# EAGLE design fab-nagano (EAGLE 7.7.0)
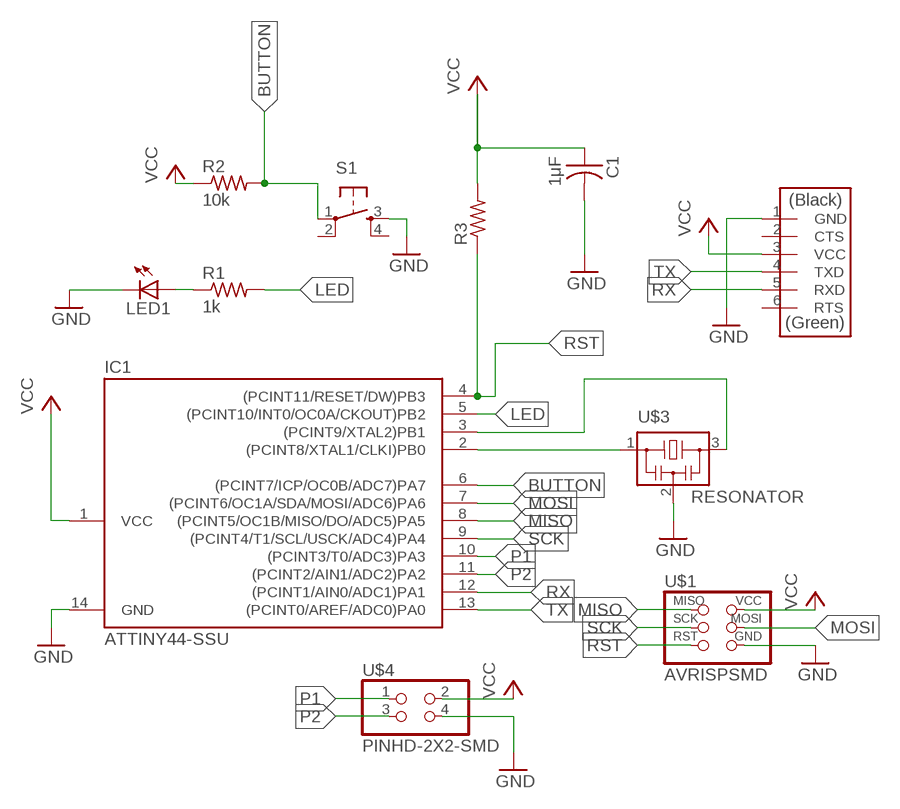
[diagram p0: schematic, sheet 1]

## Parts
C1  1μF  CAP-US1206FAB  [C1206FAB]
IC1  ATTINY44-SSU  [SOIC14]
LED1  LEDCHIP-LED0805  [CHIP-LED0805]
R1  1k  RES-US1206FAB  [R1206FAB]
R2  10k  RES-US1206FAB  [R1206FAB]
R3  RES-US1206FAB  [R1206FAB]
S1  6MM_SWITCH6MM_SWITCH  [6MM_SWITCH]
U$1  AVRISPSMD  [2X03SMD]
U$2  FTDI-SMD-HEADER  [1X06SMD]
U$3  RESONATOR  [EFOBM]
U$4  PINHD-2X2-SMD  [2X02SMD]

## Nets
BUTTON: IC1.6((PCINT7/ICP/OC0B/ADC7)PA7) R2.2 S1.1(P)
GND: C1.2 IC1.14(GND) LED1.C S1.3(S) U$1.6(GND) U$2.1(GND) U$3.2 U$4.4
LED: IC1.5((PCINT10/INT0/OC0A/CKOUT)PB2) R1.2
MISO: IC1.8((PCINT5/OC1B/MISO/DO/ADC5)PA5) U$1.1(MISO)
MOSI: IC1.7((PCINT6/OC1A/SDA/MOSI/ADC6)PA6) U$1.4(MOSI)
N$1: LED1.A R1.1
N$2: IC1.2((PCINT8/XTAL1/CLKI)PB0) U$3.1
N$3: IC1.3((PCINT9/XTAL2)PB1) U$3.3
P1: IC1.10((PCINT3/T0/ADC3)PA3) U$4.1
P2: IC1.11((PCINT2/AIN1/ADC2)PA2) U$4.3
RST: IC1.4((PCINT11/RESET/DW)PB3) R3.1 U$1.5(RST)
RX: IC1.12((PCINT1/AIN0/ADC1)PA1) U$2.5(RXD)
SCK: IC1.9((PCINT4/T1/SCL/USCK/ADC4)PA4) U$1.3(SCK)
TX: IC1.13((PCINT0/AREF/ADC0)PA0) U$2.4(TXD)
VCC: C1.1 IC1.1(VCC) R2.1 R3.2 U$1.2(VCC) U$2.3(VCC) U$4.2
Unconnected: S1.2(P1) S1.4(S1) U$2.2(CTS) U$2.6(RTS)

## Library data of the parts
C1 = fab:CAP-US
IC1 = fab:ATTINY44
LED1 = led:LED: LED
R1-R3 = fab:RES-US: Resistor (US Symbol)
S1 = fab:6MM_SWITCH: OMRON SWITCH
U$1 = fab:AVRISP
U$2 = fab:FTDI-SMD-HEADER
U$3 = fab:RESONATOR
U$4 = fab:PINHD-2X2-SMD

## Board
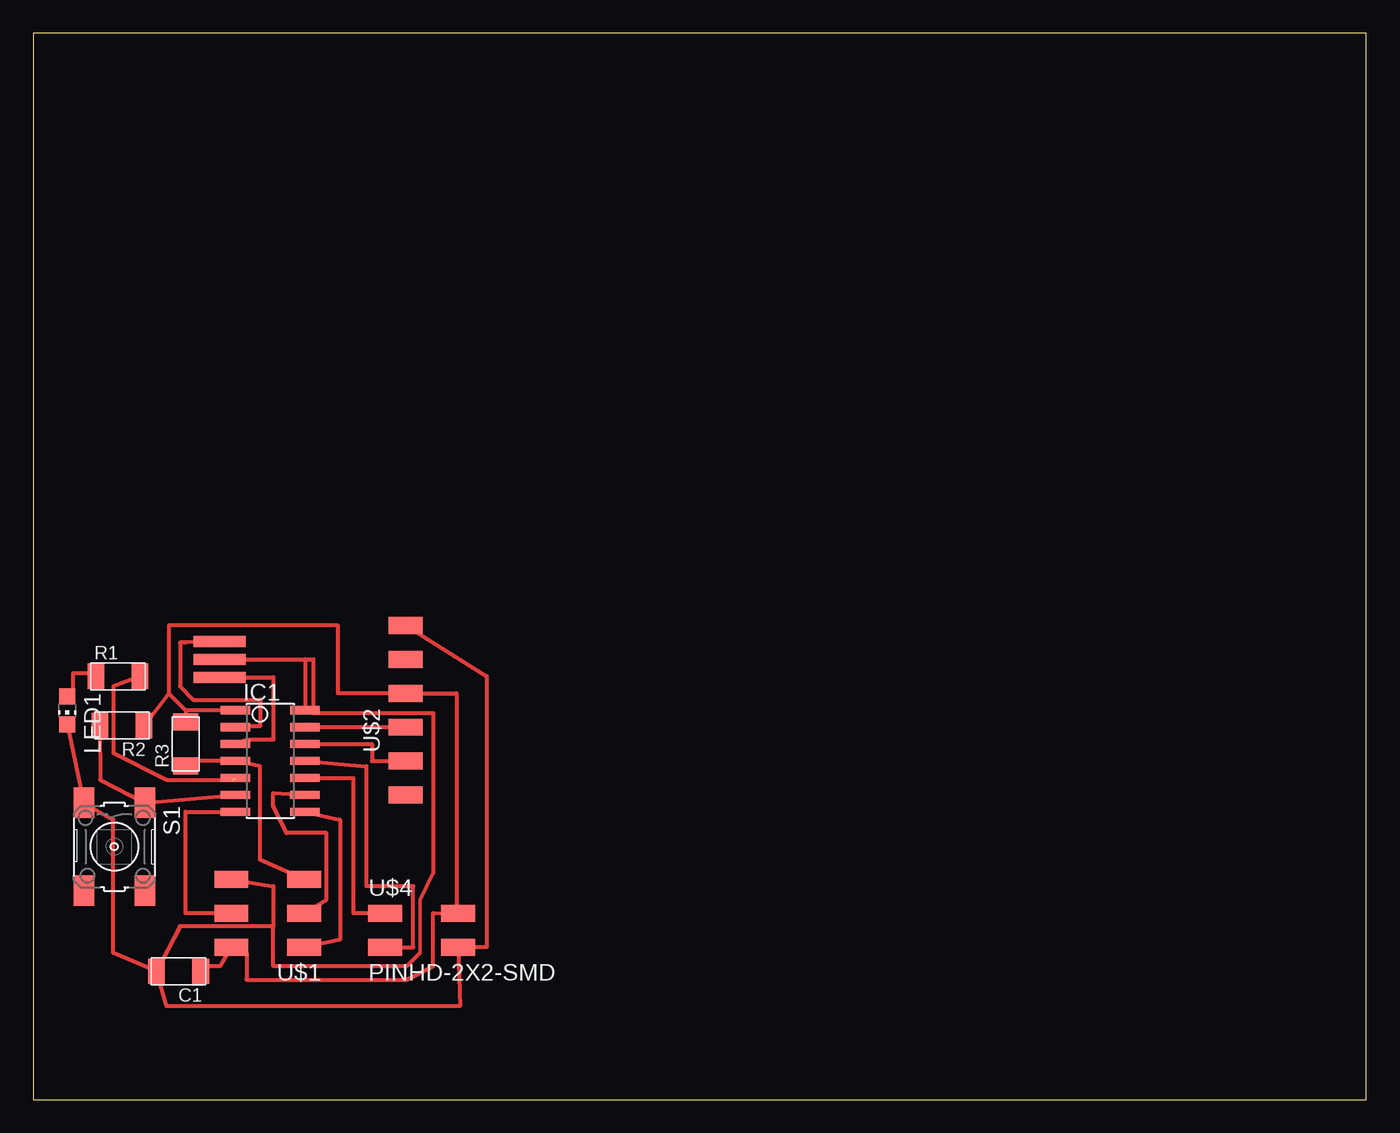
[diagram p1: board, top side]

Size 100 x 80 mm. Coordinates in mm from the lower left corner, seen from the top.
Outline: 0,0 100,0 100,80 0,80 0,0
Copper layers (1*16): Top 0.035mm / dielectric 1.5mm / Bottom 0.035mm
Design rules "default": minimum track width 10mil, minimum drill 24mil, track to track 8mil, track to pad 8mil, pad to pad 8mil, via to via 8mil, smd to smd 8mil, copper to edge 40mil, drill to drill 8mil, minimum pad ring 10mil, minimum via ring 8mil, stop-mask expansion 4mil, vias tented up to drill 0mil, thermal gap 10mil

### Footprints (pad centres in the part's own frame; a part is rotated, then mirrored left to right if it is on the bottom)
C1206FAB = smd 1.27 x 1.905: 1 -1.651,0; 2 1.651,0
SOIC14 = smd 0.61 x 2.21: 1 -3.81,-2.603; 2 -2.54,-2.603; 3 -1.27,-2.603; 4 0,-2.603; 5 1.27,-2.603; 6 2.54,-2.603; 7 3.81,-2.603; 8 3.81,2.603; 9 2.54,2.603; 10 1.27,2.603; 11 0,2.603; 12 -1.27,2.603; 13 -2.54,2.603; 14 -3.81,2.603
CHIP-LED0805 = smd 1.2 x 1.2: A 0,-1.05; C 0,1.05
R1206FAB = smd 1.27 x 1.905: 1 -1.651,0; 2 1.651,0
6MM_SWITCH = smd 2.286 x 1.524: 1 -3.302,2.286; 2 3.302,2.286; 3 -3.302,-2.286; 4 3.302,-2.286
2X03SMD = smd 2.54 x 1.27: 1 -2.54,2.54; 2 2.92,2.54; 3 -2.54,0; 4 2.92,0; 5 -2.54,-2.54; 6 2.92,-2.54
1X06SMD = smd 2.54 x 1.27: 1 0,6.35; 2 0,3.81; 3 0,1.27; 4 0,-1.27; 5 0,-3.81; 6 0,-6.35
EFOBM = smd 0.8 x 3.9: 1 -1.35,0; 2 0,0; 3 1.35,0
2X02SMD = smd 2.54 x 1.27: 1 -2.54,1.27; 2 2.92,1.27; 3 -2.54,-1.27; 4 2.92,-1.27

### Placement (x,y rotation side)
C1  10.89,9.62 180 top
IC1  17.78,25.4 270 top
LED1  2.54,29.21 180 top
R1  6.35,31.75 0 top
R2  6.65,28.06 180 top
R3  11.43,26.67 90 top
S1  6.08,18.97 270 top
U$1  17.78,13.97 180 top
U$2  27.94,29.21 0 top
U$3  13.97,33.02 270 top
U$4  28.94,12.7 0 top

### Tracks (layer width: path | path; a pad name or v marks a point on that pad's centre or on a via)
BUTTON
  Top 0.305: IC1.6 S1.1 5,24 R2.2
GND
  Top 0.254: 30,17 29,15 29,11
  Top 0.305: U$3.2 20.38,33.02 | 20.38,33.02 IC1.14 | U$2.1 34.02,31.75 34.02,11.43 U$4.4 32,7 10,7 C1.2 | C1.2 6,11 6,21 S1.3 LED1.C | U$1.6 18,16 18,13 | 18,13 11,13 C1.2 | 20.38,33.02 21,33.02 21,29 30,29 30,17 | 29,11 28,10 18,10 18,13
LED  (1 unrouted)
  Top 0.305: R1.2 6,31 6,26 10,24 15,24
MISO
  Top 0.305: IC1.8 23,21 23,12 U$1.1
MOSI
  Top 0.305: U$1.4 11.43,13.97 11.43,21.59 IC1.7
N$1
  Top 0.305: LED1.A 3,30.26 3,32 4.7,32 R1.1
N$2
  Top 0.305: U$3.1 11.43,34.29 11,34.29 11,31 12,30 17,30 17,28 16,28 IC1.2
N$3
  Top 0.305: U$3.3 18,31.67 18,27 16,27 IC1.3
P1
  Top 0.305: IC1.10 24,24.13 24,14 25.4,14 U$4.1
P2
  Top 0.305: U$4.3 28.5,11.43 28.5,16 25,16 25,25 IC1.11
RST
  Top 0.305: R3.1 11.43,25.4 IC1.4 17,25 17,18 U$1.5
RX
  Top 0.305: IC1.12 25.4,26.67 25.4,25.4 U$2.5
SCK
  Top 0.305: U$1.3 22,15 22,20 19,20 18,22 18,23 IC1.9
TX
  Top 0.305: IC1.13 U$2.4
VCC
  Top 0.305: IC1.1 11.43,29.21 | 11.43,29.21 R3.2 | 10.16,30.48 10.16,35.56 22.86,35.56 22.86,30.48 U$2.3 31.75,30.48 31.75,13.97 U$4.2 30,14 30,10 28,9 16,9 16,11 U$1.2 14,10 13,10 C1.1 | 10.16,30.48 11.43,29.21 | 10.16,30.48 R2.1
